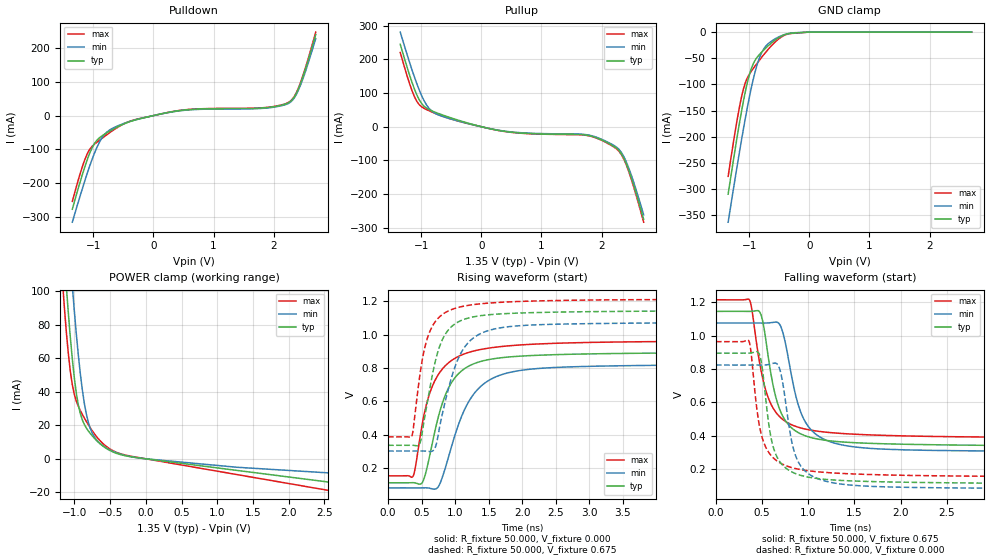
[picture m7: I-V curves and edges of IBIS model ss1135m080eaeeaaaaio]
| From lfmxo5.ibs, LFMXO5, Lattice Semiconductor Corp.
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|Model ss1135m080eaeeaaaaio
[Model] ss1135m080eaeeaaaaio
| Clamp models do not include dynamic input termination. Please refer to
| the ss1135axxxeaeeaaaain model for input termination.
Model_type I/O
Polarity   Non-Inverting
Enable   Active-Low
Vinl =  0.575V
Vinh =  0.775V
Vmeas =  0.675V
Cref =  30.000pF
Rref =  50.000
Vref =  0.675V
C_comp   5.000pF   4.000pF   5.500pF
[Temperature Range]   25.000   0.125k   -40.000
[Voltage Range]   1.350V   1.280V   1.420V
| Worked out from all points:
|   slope of the pulldown table from 0 to 0.203 V, typ, clamps not added: 25.7 ohm
|   slope of the pullup table from 0 to 0.203 V, typ, clamps not added: 24.7 ohm
|   GND clamp passes 1 mA (typ) near -0.15 V on its own axis
|   POWER clamp passes 1 mA (typ) near -0.17 V on its own axis
|   rising waveform, R_fixture 50.000, V_fixture 0.000: 20-80 % time 372ps typ, 469ps min, 375ps max; typ from 0.112 V to 0.895 V
|   rising waveform, R_fixture 50.000, V_fixture 0.675: 20-80 % time 282ps typ, 359ps min, 247ps max; typ from 0.336 V to 1.15 V
|   falling waveform, R_fixture 50.000, V_fixture 0.675: 20-80 % time 206ps typ, 235ps min, 218ps max; typ from 1.15 V to 0.336 V
|   falling waveform, R_fixture 50.000, V_fixture 0.000: 20-80 % time 150ps typ, 172ps min, 158ps max; typ from 0.895 V to 0.112 V
[Pulldown]
|Voltage   I(typ)   I(min)   I(max)
-1.35V    -276.8mA   -315.1mA   -253.5mA
-1.186V   -176.1mA   -217.7mA   -152.5mA
-1.063V   -112.3mA   -150.2mA   -100.2mA
-899mV    -65.48mA   -78.63mA   -72.91mA
-735mV    -46.76mA   -43.13mA   -51.29mA
-366mV    -16.25mA   -15.67mA   -15.03mA
331mV     12.1mA     11.5mA     12.46mA
1.807V    22.43mA    21.31mA    23.1mA
2.217V    35.4mA     33.63mA    36.46mA
2.34V     54.13mA    51.43mA    55.76mA
2.422V    83.51mA    79.33mA    86.01mA
2.7V      239.7mA    227.7mA    246.9mA
[Pullup]
|Voltage   I(typ)   I(min)   I(max)
-1.35V    245mA      281.2mA    220.6mA
-1.195V   153.6mA    191.3mA    127.9mA
-1.072V   93.9mA     126.8mA    74.67mA
-949mV    59.98mA    75.75mA    54.22mA
-826mV    47.27mA    46.49mA    43.83mA
281mV     -10.8mA    -10.26mA   -11.13mA
1.716V    -24.22mA   -23.01mA   -24.95mA
2.085V    -46.61mA   -44.28mA   -48.01mA
2.249V    -64.05mA   -60.85mA   -65.97mA
2.372V    -94.3mA    -89.6mA    -97.1mA
2.495V    -151.9mA   -144.3mA   -156.5mA
2.7V      -275.5mA   -261.7mA   -283.8mA
[GND_clamp]
|Voltage   I(typ)   I(min)   I(max)
-1.35V    -309.8mA   -363.4mA   -275.8mA
-1.21V    -207.1mA   -262.8mA   -173.9mA
-1.126V   -150.5mA   -205.1mA   -123.2mA
-1.07V    -117mA     -168.5mA   -98.8mA
-986mV    -77.25mA   -118.1mA   -78.4mA
-902mV    -53.89mA   -76.04mA   -64.81mA
-818mV    -41.42mA   -46.02mA   -52mA
-734mV    -31.56mA   -28.41mA   -39.82mA
-650mV    -22.69mA   -19.03mA   -28.57mA
-398mV    -4.585mA   -4.332mA   -5.35mA
-6mV      -40.55uA   -29.87uA   -52.89uA
2.7V      0A         0A         0A
[POWER_clamp]
|Voltage   I(typ)   I(min)   I(max)
-1.35V    264.6mA    312.3mA    234.2mA
-1.17V    138mA      188.5mA    107.5mA
-1.142V   120.1mA    170.4mA    90.88mA
-1.114V   103.1mA    152.7mA    75.88mA
-1.03V    59.59mA    103.2mA    44.19mA
-946mV    32.22mA    62.05mA    31.33mA
-890mV    23.29mA    41.28mA    26.5mA
-834mV    18.42mA    26.8mA     22.3mA
-722mV    12.33mA    13.1mA     15mA
-554mV    6.226mA    6.542mA    7.404mA
-22mV     128.8uA    103.1uA    167.9uA
2.7V      -14.6mA    -8.747mA   -19.86mA
[Ramp]
| variable   typ   min   max
dV/dt_r   0.470/0.378n   0.446/0.470n   0.486/0.381n
dV/dt_f   0.431/0.328n   0.419/0.353n   0.430/0.374n
R_load = 50.000
[Rising Waveform]
R_fixture = 50.000
V_fixture = 0.000
V_fixture_min = 0.000
V_fixture_max = 0.000
|  time   V(typ)   V(min)   V(max)
0s        111.5mV    80.89mV    153.4mV
373ps     112.2mV    80.91mV    150.8mV
527ps     126.9mV    81.29mV    501mV
737ps     487.2mV    81.61mV    752.8mV
972ps     728.2mV    364.4mV    852.2mV
1.166ns   803.1mV    571.6mV    889mV
1.377ns   839.1mV    688.3mV    911.1mV
1.847ns   867.8mV    776.7mV    934.8mV
2.71ns    882.5mV    807mV      951mV
10ns      894.5mV    823.6mV    963.5mV
[Rising Waveform]
R_fixture = 50.000
V_fixture = 0.675
V_fixture_min = 0.642
V_fixture_max = 0.710
|  time   V(typ)   V(min)   V(max)
0s        336.4mV    302.1mV    386.9mV
356ps     336.6mV    302.1mV    392.7mV
487ps     363.4mV    302.2mV    792.6mV
567ps     552mV      301.5mV    953.3mV
687ps     809.9mV    311.1mV    1.068V
847ps     998.9mV    591mV      1.131V
1.127ns   1.091V     917mV      1.171V
1.477ns   1.119V     1.022V     1.189V
2.157ns   1.132V     1.059V     1.202V
10ns      1.145V     1.075V     1.214V
[Falling Waveform]
R_fixture = 50.000
V_fixture = 0.675
V_fixture_min = 0.642
V_fixture_max = 0.710
|  time   V(typ)   V(min)   V(max)
0s        1.145V     1.075V     1.214V
362ps     1.144V     1.075V     1.214V
477ps     1.138V     1.075V     823.6mV
567ps     868.9mV    1.076V     626.6mV
680ps     573.2mV    1.074V     520mV
740ps     500.8mV    984.1mV    491.1mV
900ps     416.6mV    569.8mV    449.9mV
1.07ns    384.2mV    414.8mV    430.1mV
2.04ns    349.6mV    316.1mV    399.5mV
10ns      336.4mV    302.1mV    386.9mV
[Falling Waveform]
R_fixture = 50.000
V_fixture = 0.000
V_fixture_min = 0.000
V_fixture_max = 0.000
|  time   V(typ)   V(min)   V(max)
0s        894.5mV    823.6mV    963.5mV
356ps     894.4mV    823.4mV    967.6mV
467ps     891.1mV    823.4mV    470.3mV
587ps     416.1mV    829mV      289mV
670ps     264.1mV    824.7mV    246.3mV
720ps     225.6mV    725.6mV    230.5mV
840ps     179.1mV    320.6mV    207.1mV
970ps     156.4mV    187mV      193.3mV
1.917ns   123.6mV    93.38mV    165mV
10ns      111.5mV    80.89mV    153.4mV
